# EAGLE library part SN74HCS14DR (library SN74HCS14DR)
Inverters Hex inverter with Schmitt-trigger inputs Source: Datasheet
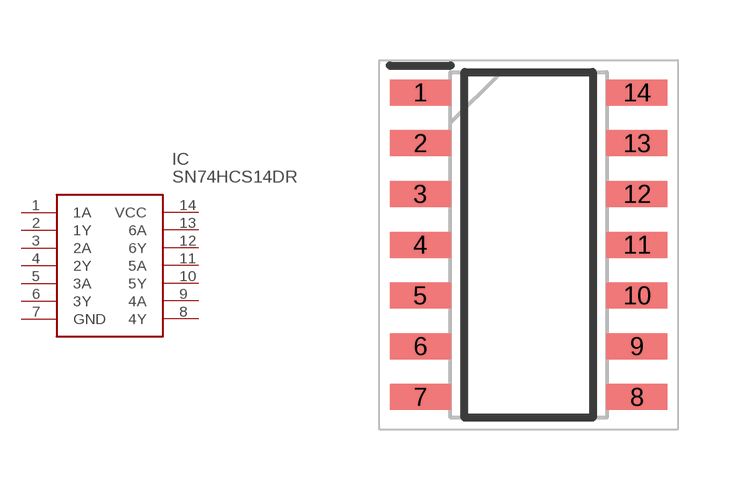
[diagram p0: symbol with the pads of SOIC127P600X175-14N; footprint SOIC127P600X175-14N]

Designator prefix IC

## SN74HCS14DR (Description: Inverters Hex inverter with Schmitt-trigger inputs; Height: 1.75mm; Manufacturer_Name: Texas Instruments; Manufacturer_Part_Number: SN74HCS14DR; Mouser_Part_Number: 595-SN74HCS14DR; Mouser_Price-Stock: https://www.mouser.co.uk/ProductDetail/Texas-Instruments/SN74HCS14DR?qs=sPbYRqrBIVmUkCpweRJJCA%3D%3D)  [SOIC127P600X175-14N]
1  1A
2  1Y
3  2A
4  2Y
5  3A
6  3Y
7  GND  pwr
8  4Y
9  4A
10  5Y
11  5A
12  6Y
13  6A
14  VCC  pwr

## Footprint SOIC127P600X175-14N (pad centres in mm)
14 Ld SOIC
smd 1.525 x 0.65: 1 -2.712,3.81; 2 -2.712,2.54; 3 -2.712,1.27; 4 -2.712,0; 5 -2.712,-1.27; 6 -2.712,-2.54; 7 -2.712,-3.81; 8 2.712,-3.81; 9 2.712,-2.54; 10 2.712,-1.27; 11 2.712,0; 12 2.712,1.27; 13 2.712,2.54; 14 2.712,3.81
